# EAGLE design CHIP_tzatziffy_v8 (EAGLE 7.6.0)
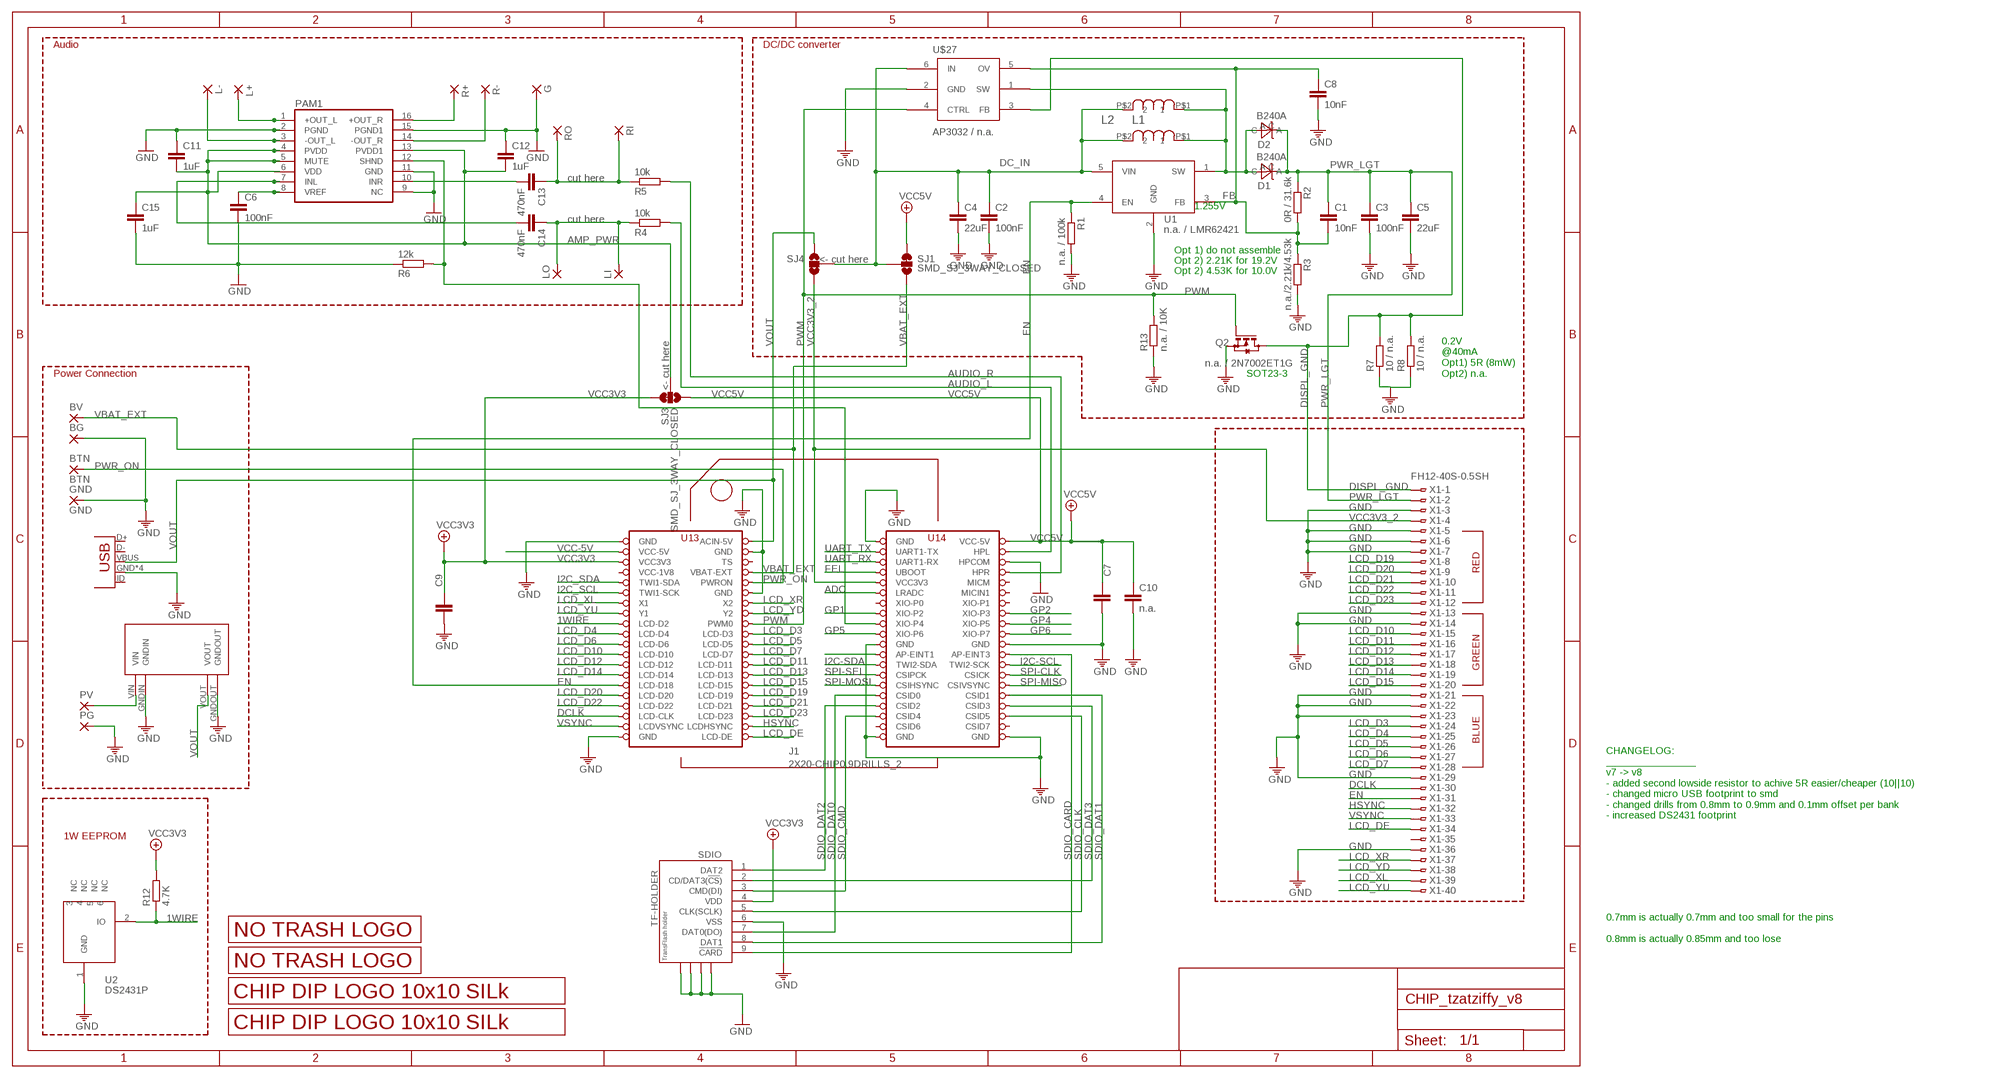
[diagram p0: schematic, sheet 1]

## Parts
BG  1,6/0,8  [1,6/0,8]
BTN  BTN  SMD2  [SMD1,27-2,54]
BV  1,6/0,8  [1,6/0,8]
C1  10nF  C-EUC0805  [C0805]
C2  100nF  C-EUC0805  [C0805]
C3  100nF  C-EUC0805  [C0805]
C4  22uF  C-EUC1206  [C1206]
C5  22uF  C-EUC1206  [C1206]
C6  100nF  C-EUC0805  [C0805]
C7  n.a.  C-EUC0805  [C0805]
C8  10nF  C-EUC0805  [C0805]
C9  n.a.  C-EUC0805  [C0805]
C10  n.a.  C-EUC0805  [C0805]
C11  1uF  C-EUC0805  [C0805]
C12  1uF  C-EUC0805  [C0805]
C13  470nF  C-EUC0805  [C0805]
C14  470nF  C-EUC0805  [C0805]
C15  1uF  C-EUC0805  [C0805]
D1  B240A  DIODE_SCHTKY_B240  [DO-214AC]
D2  B240A  DIODE_SCHTKY_B240  [DO-214AC]
G  1,6/0,8  [1,6/0,8]
GND  GND  SMD2  [SMD1,27-2,54]
J1  2X20-CHIP0.9DRILLS_2  [2X20CHIP_BANK_OFFSET_TH_0.9]
JP1  USBMICRO_SMD  [USB-B-MICRO-SMD_V03]
L1  SRN6045-100M  [SRN6045]
L2  SRN6045-100M  [SRN6045]
L+  1,6/0,8  [1,6/0,8]
L-  1,6/0,8  [1,6/0,8]
LI  1,6/0,8  [1,6/0,8]
LO  1,6/0,8  [1,6/0,8]
PAM1  PAM8403  [SOP-16]
PG  1,6/0,8  [1,6/0,8]
PV  1,6/0,8  [1,6/0,8]
Q2  n.a. / 2N7002ET1G  BSS123  [SOT23]
R1  n.a. / 100k  R-EU_M0805  [M0805]
R2  0R / 31.6k  R-EU_M0805  [M0805]
R3  n.a./2.21k/4.53k  R-EU_M0805  [M0805]
R4  10k  R-EU_R0805  [R0805]
R5  10k  R-EU_R0805  [R0805]
R6  12k  R-EU_R0805  [R0805]
R7  10 / n.a.  R-EU_M0805  [M0805]
R8  10 / n.a.  R-EU_M0805  [M0805]
R12  4.7K  R-EU_M0805  [M0805]
R13  n.a. / 10K  R-EU_M0805  [M0805]
R+  1,6/0,8  [1,6/0,8]
R-  1,6/0,8  [1,6/0,8]
RI  1,6/0,8  [1,6/0,8]
RO  1,6/0,8  [1,6/0,8]
SDIO  TF-HOLDER  [TF-PULL]
SJ1  SMD_SJ_3WAY_CLOSED  [SMD_SJ_3WAY_CLOSED]
SJ3  SMD_SJ_3WAY_CLOSED  [SMD_SJ_3WAY_CLOSED]
SJ4  SMD_SJ_3WAY_OPENT  [SMD_SJ_3WAY_OPEN]
U1  n.a. / LMR62421  LMR62421  [SOT23-5]
U2  DS2431P  [TSOC6]
U$2  LOGO_10X10_SILK  [LOGO2_10X10_SILK]
U$3  LOGO_NO_TRASHROHS  [LOGO_ROHS_SYM]
U$4  LOGO_NO_TRASHNO_TRASH  [LOGO_ROHS_NO_TRASH]
U$5  LOGO_10X10_SILK  [LOGO2_10X10_SILK]
U$10  MP1584EN_FRAMELESS  [MP1584EN_FRAMELESS]
U$27  AP3032 / n.a.  AP3032  [SOT23-6]
X1  FH12-40S-0.5SH  [FH12-40S-0.5SH]

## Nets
1WIRE: J1.LCD-D2 R12.1 U2.2(IO)
ADC: J1.LRADC
AMP_PWR: C11.2 C12.2 C15.1 PAM1.4(PVDD) PAM1.5(MUTE) PAM1.6(VDD) PAM1.13(PVDD1) SJ3.2
AUDIO_L: J1.HPL R4.2
AUDIO_R: J1.HPR R5.2
DC_IN: C2.1 C4.1 L1.P$2 L2.P$2 SJ1.2 SJ4.2 U1.5(VIN) U$27.6(IN)
DCLK: J1.LCD-CLK X1.30
DISPL_GND: Q2.3(D) R7.2 R8.2 U$27.3(FB) X1.1
EN: J1.LCD-D18 R1.1 U1.4(EN) X1.31
FB: C1.2 C8.1 R2.2 R3.1 U1.3(FB) U$27.5(OV)
FEL: J1.FEL(UBOOT)
GND: BG.1(P) C2.2 C3.2 C4.2 C5.2 C6.2 C7.2 C8.2 C9.2 C10.2 C11.1 C12.1 C15.2 G.1(P) GND.1(P) J1.GND@1(GND) J1.GND@2(GND) J1.GND@3(GND) J1.GND@4(GND) J1.GND@5(GND) J1.GND@6(GND) J1.GND@7(GND) J1.GND@8(GND) J1.GND@10(GND) J1.HPCOM JP1.GND JP1.SHIELD1(GND) JP1.SHIELD2(GND) JP1.SHIELD3(GND) PAM1.2(PGND) PAM1.9(NC) PAM1.11(GND) PAM1.15(PGND1) PG.1(P) Q2.2(S) R1.2 R3.2 R6.1 R7.1 R8.1 R13.1 SDIO.6(VSS) SDIO.S1 SDIO.S2 SDIO.S3 SDIO.S4 U1.2(GND) U2.1(GND) U$10.GNDIN U$10.GNDOUT U$27.2(GND) X1.3 X1.5 X1.6 X1.7 X1.13 X1.14 X1.21 X1.22 X1.23 X1.29 X1.36
GP1: J1.XIO-P2
GP2: J1.XIO-P3
GP3: J1.XIO-P4 PAM1.12(SHND) R6.2
GP4: J1.XIO-P5
GP5: J1.XIO-P6
GP6: J1.XIO-P7
HSYNC: J1.LCD-HSYNC(LCDHSYNC) X1.32
I2C-SCL: J1.TWI2-SCK
I2C-SDA: J1.TWI2-SDA
I2C_SCL: J1.TWI1-SCK
I2C_SDA: J1.TWI1-SDA
INL: C14.2 PAM1.7(INL)
INR: C13.2 PAM1.10(INR)
KPD_INT: J1.AP-EINT1
L+OUT: L+.1(P) PAM1.1(+OUT_L)
L-OUT: L-.1(P) PAM1.3(-OUT_L)
LCD_D3: J1.LCD-D3 X1.24
LCD_D4: J1.LCD-D4 X1.25
LCD_D5: J1.LCD-D5 X1.26
LCD_D6: J1.LCD-D6 X1.27
LCD_D7: J1.LCD-D7 X1.28
LCD_D10: J1.LCD-D10 X1.15
LCD_D11: J1.LCD-D11 X1.16
LCD_D12: J1.LCD-D12 X1.17
LCD_D13: J1.LCD-D13 X1.18
LCD_D14: J1.LCD-D14 X1.19
LCD_D15: J1.LCD-D15 X1.20
LCD_D19: J1.LCD-D19 X1.8
LCD_D20: J1.LCD-D20 X1.9
LCD_D21: J1.LCD-D21 X1.10
LCD_D22: J1.LCD-D22 X1.11
LCD_D23: J1.LCD-D23 X1.12
LCD_DE: J1.LCD-DE X1.34
LCD_XL: J1.X1 X1.39
LCD_XR: J1.X2 X1.37
LCD_YD: J1.Y2 X1.38
LCD_YU: J1.Y1 X1.40
N$38: C6.1 PAM1.8(VREF)
N$41: C14.1 LI.1(P) LO.1(P) R4.1
N$43: C13.1 R5.1 RI.1(P) RO.1(P)
PWM: J1.PWM0 Q2.1(G) R13.2 U$27.4(CTRL)
PWR_IN: PV.1(P) U$10.VIN
PWR_LGT: C1.1 C3.1 C5.1 D1.C D2.C R2.1 X1.2
PWR_ON: BTN.1(P) J1.PWRON
R+OUT: PAM1.16(+OUT_R) R+.1(P)
R-OUT: PAM1.14(-OUT_R) R-.1(P)
SDIO_CARD: J1.AP-EINT3 SDIO.9(!CARD)
SDIO_CLK: J1.CSID5 SDIO.5(CLK(SCLK))
SDIO_CMD: J1.CSID4 SDIO.3(CMD(DI))
SDIO_DAT0: J1.CSID0 SDIO.7(DAT0(DO))
SDIO_DAT1: J1.CSID1 SDIO.8(DAT1)
SDIO_DAT2: J1.CSID2 SDIO.1(DAT2)
SDIO_DAT3: J1.CSID3 SDIO.2(CD/DAT3(!CS!))
SPI-CLK: J1.CSICK
SPI-MISO: J1.CSIVSYNC
SPI-MOSI: J1.CSIHSYNC
SPI-SEL: J1.CSIPCK
UART_RX: J1.UART1-RX
UART_TX: J1.UART1-TX
VBAT_EXT: BV.1(P) J1.BAT(VBAT-EXT) SJ1.3
VCC3V3: C9.1 J1.VCC3V3 R12.2 SDIO.4(VDD) SJ3.1
VCC3V3_2: J1.VCC3V3@1(VCC3V3) SJ4.3 X1.4
VCC5V: C7.1 C10.1 J1.VCC5V@1(VCC-5V) SJ1.1 SJ3.3
VCC-5V: J1.VCC5V@0(VCC-5V)
VOUT: J1.CHG-IN(ACIN-5V) JP1.VBUS SJ4.1 U$10.VOUT
VREG_OUTPUT: D1.A D2.A L1.P$1 L2.P$1 U1.1(SW) U$27.1(SW)
VSYNC: J1.LCD-VSYNC(LCDVSYNC) X1.33
Unconnected: J1.CSID6 J1.CSID7 J1.MICIN1 J1.MICM J1.TS J1.XIO-P0 J1.XIO-P1 JP1.D+ JP1.D- JP1.ID U2.3(NC) U2.4(NC) U2.5(NC) U2.6(NC) X1.35

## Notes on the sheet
- Audio | DC/DC converter
- cut here
- 1.255V
- cut here
- Opt 1) do not assemble
- <- cut here | Opt 2) 2.21K for 19.2V
- Opt 2) 4.53K for 10.0V
- <- cut here
- Power Connection | SOT23-3
- 0.2V
  @40mA
  Opt1) 5R (8mW)
  Opt2) n.a.
- RED
- GREEN
- BLUE
- CHANGELOG:
  _______________
  v7 -> v8
  - added second lowside resistor to achive 5R easier/cheaper (10||10)
  - changed micro USB footprint to smd
  - changed drills from 0.8mm to 0.9mm and 0.1mm offset per bank
  - increased DS2431 footprint
- 1W EEPROM
- 0.7mm is actually 0.7mm and too small for the pins
  
  0.8mm is actually 0.85mm and too lose

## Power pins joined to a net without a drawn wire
VCC-1V8: J1.VCC1V8(VCC-1V8)

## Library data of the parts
BG BV G L+ L- LI LO PG PV R+ R- RI RO = wirepad:1,6/0,8: THROUGH-HOLE PAD
BTN GND = wirepad:SMD2: SMD PAD
C1-C15 = rcl:C-EU: CAPACITOR, European symbol
D1 D2 = Keyboard v0_5:DIODE_SCHTKY_B240; DESCRIPTION: DIODE SMD General Purpose 400V 1A 1.4W RoHS DO-214AC; FOOTPRINT: DO-214AC; LINK: http://www.digikey.com/product-detail/en/B240A-13-F/B240A-FDICT-ND/717810; MFG: DIGIKEY; MFG_PN: B240A-FDICT-ND; PART_TYPE: DIODE; PRICE: 0.11; VENDOR: DIODES; VENDOR_PART_NUMBER: B240A-13-F
J1 = JKW_CHIP:2X20-CHIP: Chip header; DESC: 0.9mm drills, moved outer rows 0.1mm towards outside, inner rows 0.1mm inwards
JP1 = JKW_CHIP:USB
L1 L2 = Keyboard v0_5:SRN6045-100M; DESCRIPTION: power inductor 10uH 2.5A 58.6 mohm; FOOTPRINT: SRN6045; LINK: http://www.digikey.com/product-detail/en/SRN6045-100M/SRN6045-100MTR-ND/2756120; MFG: DIGIKEY; MFG_PN: SRN6045-100MTR-ND; PART_TYPE: IND; PRICE: 0.15; TOLLERANCE: ±20%; VENDOR: BOURNS; VENDOR_PART_NUMBER: SRN6045-100M
PAM1 = JKW_CHIP:PAM8403: Dual channel audio amplifier IC - PAM8403
Q2 = transistor-small-signal:BSS123: N-CHANNEL MOS FET
R1-R8 R12 R13 = rcl:R-EU_: RESISTOR, European symbol
SDIO = JKW_CHIP:TF-HOLDER: TF / Micro SD socket is PUSH-PUSH type, the card can be pushed into and auto locked and pushed out by simply press the card. Surface Mounting type.
SJ1 SJ3 = JKW_CHIP:SMD_SJ_3WAY_CLOSED
SJ4 = JKW_CHIP:SMD_SJ_3WAY_OPEN: Solder Jumper 2 way solder jumper
U1 = PocketCHIP-Components-v0.7:LMR62421; DESCRIPTION: dc/dc step up, 2.1A, 1.6mhz, SOT-23-5; FOOTPRINT: SOT23-5; LINK: http://www.digikey.com/product-detail/en/LMR62421XMFE%2FNOPB/LMR62421XMFE%2FNOPBCT-ND/2777085; MFG: DIGIKEY; MFG_PN: LMR62421XMFE/NOPBCT-ND; PART_TYPE: IC; PRICE: 0.8; VENDOR: TEXAS INSTRUMENTS; VENDOR_PART_NUMBER: LMR62421XMFE/NOPB
U2 = JKW_CHIP:DS2431: 1024-Bit EEPROM This chip provides a 4x256 Bit EEPROM, which can be programmed@5V. Write protection and OTP emulation are available, too. Author: Jan Kandziora <jjj@gmx.de>; DESCRIPTION: IC, 1024-Bit, 1-Wire EEPROM, TSOC6; FOOTPRINT: TSOC6; LINK: http://www.digikey.com/product-detail/en/DS2431P%2BT%26R/DS2431P%2BT%26RCT-ND/3647900; MFG: DIGIKEY; MFG_PN: DS2431P+T&RCT-ND; PART_TYPE: IC; PRICE: 0.98; VENDOR: MAXIM; VENDOR_PART_NUMBER: DS2431P+T&R
U$2 U$5 = JKW_CHIP:LOGO_10X10_SILK
U$3 U$4 = JKW_CHIP:LOGO_NO_TRASH
U$10 = JKW_CHIP:MP1584EN_FRAMELESS
U$27 = JKW_CHIP:AP3032
X1 = Keyboard v0_5:FH12-40S-0.5S: 0.5mm Pitch Connectors For FPC/FFC Source: Data sheet; DESCRIPTION: CON ffc smd, bottom contact 40pos, 0.50mm R/A; FOOTPRINT: FH12-40S-0.5SH; LINK: http://www.digikey.com/product-detail/en/FH12-40S-0.5SH(55)/HFJ140CT-ND/1110388; MFG: DIGIKEY; MFG_PN: HFJ140CT-ND; VENDOR: HIROSE; VENDOR_PART_NUMBER: FH12-40S-0.5SH(55)

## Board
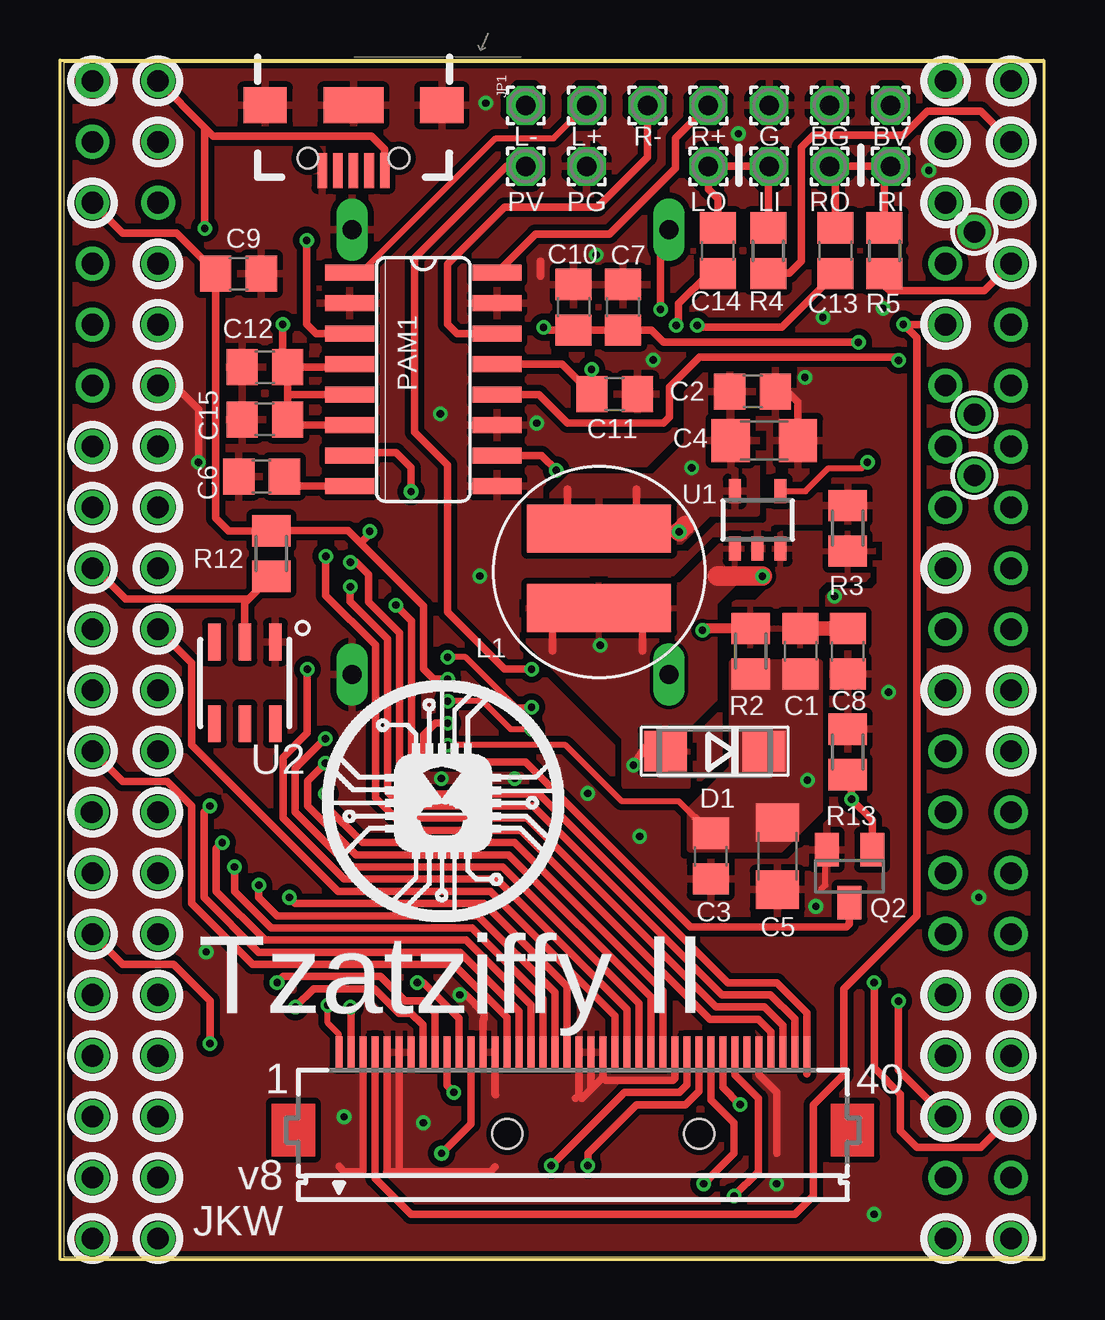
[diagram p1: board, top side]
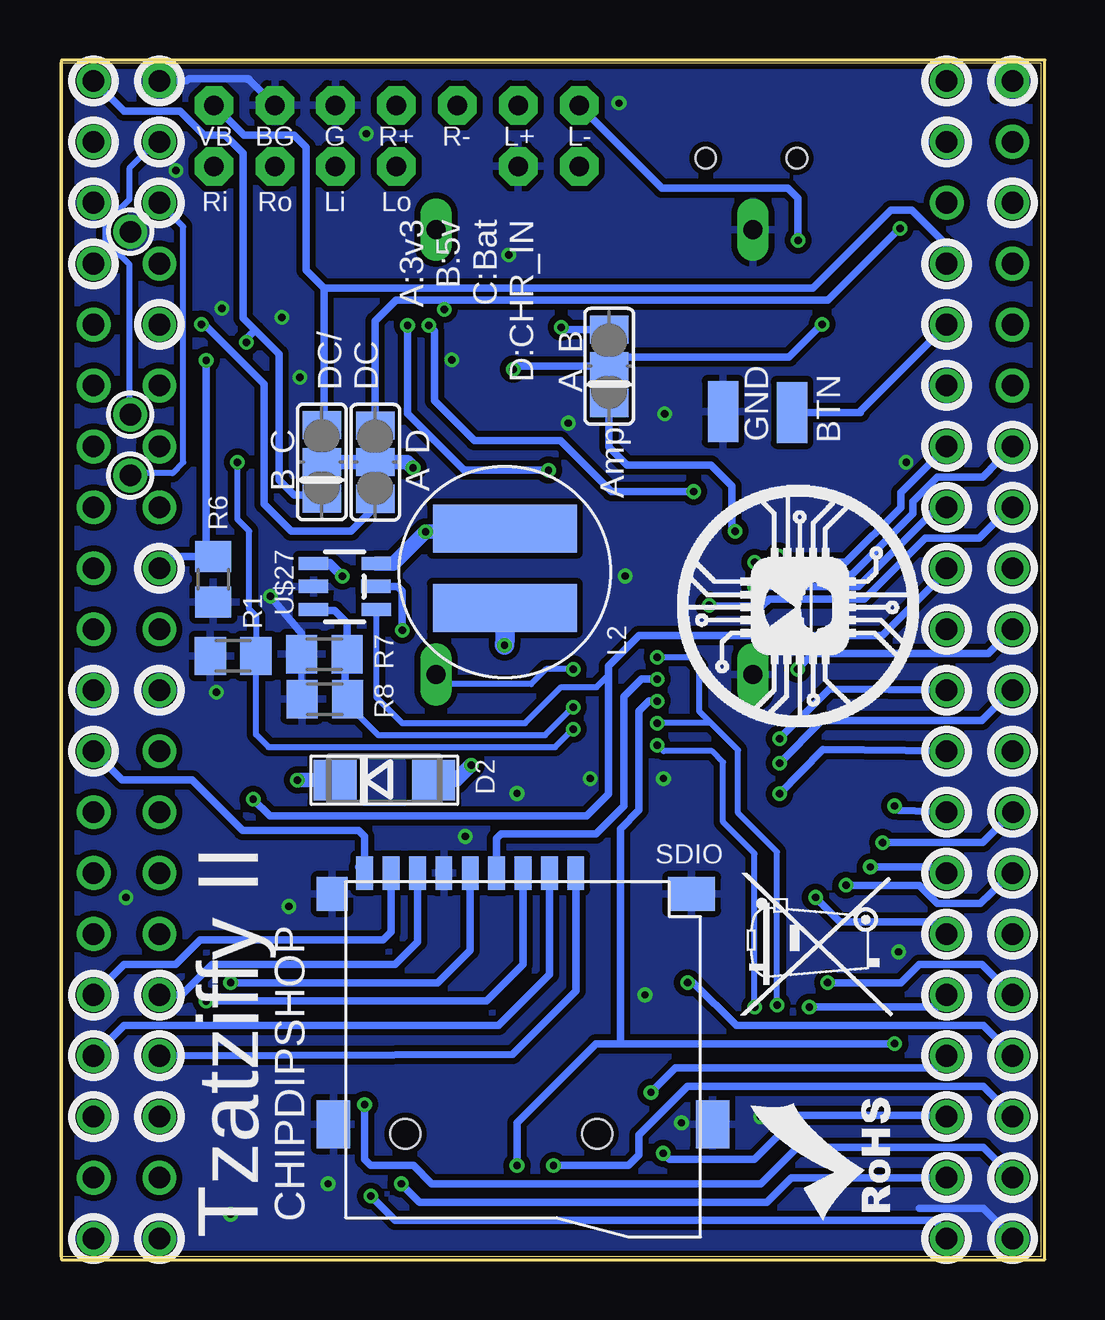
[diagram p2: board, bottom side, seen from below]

Size 41.05 x 50 mm. Coordinates in mm from the lower left corner, seen from the top.
Outline: 0.16,0.11 41.05,0.11 41.05,49.89 0.16,49.89 0.16,0.11
Copper layers (1*16): Top 0.035mm / dielectric 1.5mm / Bottom 0.035mm
Design rules "SeeedStudio_2layer_DRU_no_angle_20140221": minimum track width 6mil, minimum drill 12mil, track to track 6mil, track to pad 6mil, pad to pad 6mil, via to via 6mil, smd to smd 0mil, copper to edge 10mil, drill to drill 10mil, minimum pad ring 10mil, minimum via ring 6mil, stop-mask expansion 2mil, vias tented up to drill 100mil, thermal gap 10mil

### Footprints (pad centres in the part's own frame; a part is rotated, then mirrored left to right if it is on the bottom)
1,6/0,8 = drill 0.813 pad 1.6 octagon: 1 0,0
SMD1,27-2,54 = smd 1.27 x 2.54: 1 0,0
C0805 = smd 1.3 x 1.5: 1 -0.95,0; 2 0.95,0
C1206 = smd 1.6 x 1.8: 1 -1.4,0; 2 1.4,0
DO-214AC = smd 1.8 x 1.7: A 2.05,0; C -2.05,0
2X20CHIP_BANK_OFFSET_TH_0.9 = drill 0.9: AP-EINT1 15.14,-3.81; AP-EINT3 17.88,-3.81; BAT -17.68,16.51; CHG-IN -17.68,24.13; CSICK 17.88,-8.89; CSID0 15.14,-13.97; CSID1 17.88,-13.97; CSID2 15.14,-16.51; CSID3 17.88,-16.51; CSID4 15.14,-19.05; CSID5 17.88,-19.05; CSID6 15.14,-21.59; CSID7 17.88,-21.59; CSIHSYNC 15.14,-11.43; CSIPCK 15.14,-8.89; CSIVSYNC 17.88,-11.43; FEL 15.14,16.51; GND@1 -17.68,11.43; GND@2 -20.42,-24.13; GND@4 17.88,-1.27; GND@5 17.88,-24.13; GND@6 15.14,-24.13; GND@7 15.14,-1.27; GND@10 -17.68,21.59; HPCOM 17.88,19.05; HPL 17.88,21.59; HPR 17.88,16.51; LCD-CLK -20.42,-19.05; LCD-D2 -20.42,3.81; LCD-D3 -17.68,1.27; LCD-D4 -20.42,1.27; LCD-D5 -17.68,-1.27; LCD-D6 -20.42,-1.27; LCD-D7 -17.68,-3.81; LCD-D10 -20.42,-3.81; LCD-D11 -17.68,-6.35; LCD-D12 -20.447,-6.35; LCD-D13 -17.68,-8.89; LCD-D14 -20.42,-8.89; LCD-D15 -17.68,-11.43; LCD-D18 -20.42,-11.43; LCD-D19 -17.68,-13.97; LCD-D20 -20.42,-13.97; LCD-D21 -17.68,-16.51; LCD-D22 -20.42,-16.51; LCD-D23 -17.68,-19.05; LCD-DE -17.68,-24.13; LCD-HSYNC -17.68,-21.59; LCD-VSYNC -20.42,-21.59; LRADC 15.14,11.43; MICIN1 17.88,11.43; MICM 17.88,13.97; PWM0 -17.68,3.81; PWRON -17.68,13.97; TS -17.68,19.05; TWI1-SCK -20.42,11.43; TWI1-SDA -20.42,13.97; TWI2-SCK 17.88,-6.35; TWI2-SDA 15.14,-6.35; UART1-RX 15.14,19.05; UART1-TX 15.14,21.59; VCC1V8 -20.42,16.51; VCC3V3 -20.42,19.05; VCC3V3@1 15.14,13.97; VCC5V@0 -20.42,21.59; VCC5V@1 17.88,24.13; X1 -20.42,8.89; X2 -17.68,8.89; XIO-P0 15.14,8.89; XIO-P1 17.88,8.89; XIO-P2 15.14,6.35; XIO-P3 17.88,6.35; XIO-P4 15.14,3.81; XIO-P5 17.88,3.81; XIO-P6 15.14,1.27; XIO-P7 17.88,1.27; Y1 -20.42,6.35; Y2 -17.68,6.35 | drill 0.9 square: GND@3 -20.42,24.13; GND@8 15.14,24.13
USB-B-MICRO-SMD_V03 = smd 1.45 x 0.4: D+ 2.725,0; D- 2.725,0.65; GND 2.725,-1.3; ID 2.725,-0.65; VBUS 2.725,1.3 | smd 1.5 x 1.8: SHIELD1 0,3.685; SHIELD2 0,-3.685 | smd 1.5 x 2.5: SHIELD3 0,0 | hole 0.85: 2.2,1.9; 2.2,-1.9
SRN6045 = smd 2 x 6: P$1 1.5,0; P$2 -1.8,0
SOP-16 = smd 0.66 x 2.032: 1 -4.445,-3.073; 2 -3.175,-3.073; 3 -1.905,-3.073; 4 -0.635,-3.073; 5 0.635,-3.073; 6 1.905,-3.073; 7 3.175,-3.073; 8 4.445,-3.073; 9 4.445,3.073; 10 3.175,3.073; 11 1.905,3.073; 12 0.635,3.073; 13 -0.635,3.073; 14 -1.905,3.073; 15 -3.175,3.073; 16 -4.445,3.073
SOT23 = smd 1 x 1.4: 1 -0.95,-1.1; 2 0.95,-1.1; 3 0,1.1
M0805 = smd 1.3 x 1.6: 1 -0.95,0; 2 0.95,0
R0805 = smd 1.3 x 1.5: 1 -0.95,0; 2 0.95,0
TF-PULL = smd 0.7 x 1.4: 1 -2.2,-7.62; 2 -1.1,-7.62; 3 0,-7.62; 4 1.1,-7.62; 5 2.2,-7.62; 6 3.3,-7.62; 7 4.4,-7.62; 8 5.5,-7.62; 9 6.6,-7.62 | smd 1.4 x 2: S1 -7.9,2.85; S2 7.9,2.85 | smd 1.28 x 1.4: S3 7.96,-6.75 | smd 1.95 x 1.4: S4 -7.025,-6.75 | hole 1.25: -3.1,3.25; 4.9,3.25
SMD_SJ_3WAY_CLOSED = smd 1.168 x 1.6: 1 -1.524,0; 2 0,0; 3 1.524,0
SMD_SJ_3WAY_OPEN = smd 1.168 x 1.6: 1 -1.524,0; 2 0,0; 3 1.524,0
SOT23-5 = smd 0.5 x 1: 1 -0.95,-1.2; 2 0,-1.2; 3 0.95,-1.2; 4 0.95,1.2; 5 -0.95,1.2
TSOC6 = smd 0.53 x 1.53: 1 -1.27,-1.7; 2 0,-1.7; 3 1.27,-1.7; 4 1.27,1.7; 5 0,1.7; 6 -1.27,1.7
MP1584EN_FRAMELESS = drill 0.8 long: GNDIN 1.778,14.986; GNDOUT 20.32,14.986; VIN 1.778,1.778; VOUT 20.32,1.778
SOT23-6 = smd 0.559 x 1.219: 1 -0.95,-1.3; 2 0,-1.3; 3 0.965,-1.3; 4 0.965,1.321; 5 0,1.3; 6 -0.95,1.321
FH12-40S-0.5SH = smd 0.3 x 1.3: 1 -9.75,3.25; 2 -9.25,3.25; 3 -8.75,3.25; 4 -8.25,3.25; 5 -7.75,3.25; 6 -7.25,3.25; 7 -6.75,3.25; 8 -6.25,3.25; 9 -5.75,3.25; 10 -5.25,3.25; 11 -4.75,3.25; 12 -4.25,3.25; 13 -3.75,3.25; 14 -3.25,3.25; 15 -2.75,3.25; 16 -2.25,3.25; 17 -1.75,3.25; 18 -1.25,3.25; 19 -0.75,3.25; 20 -0.25,3.25; 21 0.25,3.25; 22 0.75,3.25; 23 1.25,3.25; 24 1.75,3.25; 25 2.25,3.25; 26 2.75,3.25; 27 3.25,3.25; 28 3.75,3.25; 29 4.25,3.25; 30 4.75,3.25; 31 5.25,3.25; 32 5.75,3.25; 33 6.25,3.25; 34 6.75,3.25; 35 7.25,3.25; 36 7.75,3.25; 37 8.25,3.25; 38 8.75,3.25; 39 9.25,3.25; 40 9.75,3.25

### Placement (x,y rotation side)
BG  32.09,48.11 0 top
BTN  10.54,35.31 180 bottom
BV  34.63,48.11 0 top
C1  30.87,25.36 90 top
C2  28.87,36.18 0 top
C3  27.13,16.82 270 top
C4  29.36,34.14 0 top
C5  29.91,16.82 270 top
C6  8.41,32.64 180 top
C7  23.47,39.7 90 top
C8  32.83,25.36 270 top
C9  7.45,41.09 0 top
C10  21.41,39.7 90 top
C11  23.13,36.07 180 top
C12  8.54,37.19 0 top
C13  32.33,42.05 270 top
C14  27.42,42.05 270 top
C15  8.54,35.02 180 top
D1  27.29,21.18 180 top
D2  27.54,19.98 0 bottom
G  29.57,48.11 0 top
GND  13.41,35.35 180 bottom
J1  21.77,25 0 top
JP1  12.23,48.11 270 top
L1  22.48,28.66 270 top
L2  22.51,28.66 270 bottom
L+  21.95,48.11 0 top
L-  19.41,48.11 0 top
LI  29.57,45.57 0 top
LO  27.03,45.57 0 top
PAM1  15.15,36.68 270 top
PG  21.95,45.57 0 top
PV  19.41,45.57 0 top
Q2  32.91,15.98 180 top
R1  33.83,25.16 180 bottom
R2  28.79,25.36 90 top
R3  32.83,30.48 90 top
R4  29.53,42.05 270 top
R5  34.37,42.05 270 top
R6  34.66,28.36 90 bottom
R7  30.04,25.23 0 bottom
R8  30.01,23.36 0 bottom
R12  8.81,29.43 90 top
R13  32.83,21.16 270 top
R+  27.03,48.11 0 top
R-  24.49,48.11 0 top
RI  34.63,45.57 0 top
RO  32.09,45.57 0 top
SDIO  21.75,8.49 180 bottom
SJ1  30.14,33.25 90 bottom
SJ3  18.16,37.23 90 bottom
SJ4  27.91,33.23 270 bottom
U1  29.08,30.83 0 top
U2  7.71,24.04 180 top
U$2  10.95,14.08 0 top
U$3  6.37,1.19 90 bottom
U$4  6.33,10.13 90 bottom
U$5  5.26,22.21 90 bottom
U$10  27.16,22.61 90 top
U$27  29.19,28.06 270 bottom
X1  21.38,5.39 0 top

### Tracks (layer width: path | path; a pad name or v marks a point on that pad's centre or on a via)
1WIRE
  Top 0.305: 7.87,27.54 2.74,27.54 1.47,28.81 J1.LCD-D2 | 7.87,27.54 R12.1 | 7.87,27.54 7.71,27.37 U2.2
AMP_PWR  (via drill 0.3)
  Top 0.305: 9.62,37.32 C12.2 | PAM1.6 10.13,34.78 C15.1 9.49,35.98 | C12.2 9.49,35.98 | PAM1.4 11.95,37.19 C12.2 | v9.29,38.98 9.29,37.4 C12.2 | 18.18,37.36 PAM1.13 20.93,37.32 C11.2 21.78,35.85 22.16,36.23 v22.16,37.11 | PAM1.5 9.56,36.05 9.49,35.98
  Bottom 0.305: v9.29,38.98 10.66,37.61 17.79,37.61 SJ3.2 22.04,37.23 v22.16,37.11
AUDIO_L
  Top 0.305: 29.16,40.98 29.15,40.99 R4.2 29.16,41.11 30.41,41.11 30.91,41.61 30.91,46.36 31.41,46.86 35.16,46.86 36.16,47.86 38.38,47.86 J1.HPL
AUDIO_R
  Top 0.305: R5.2 34.35,40.61 34.58,40.38 38.52,40.38 J1.HPR
DC_IN  (via drill 0.3)
  Top 0.305: 21.16,32.11 21.16,31.11 | 24.04,32.11 24.04,31.11
  Top 0.813: v25.81,30.33 26.07,30.59
  Bottom 0.61: 22.68,29.88 22.48,30.08 22.51,30.08 L2.P$2 22.64,30.33 v25.81,30.33 27.14,29.01 U$27.6 | SJ1.2 27.93,33.25 | 27.93,33.25 SJ4.2 | 27.93,33.25 26.58,33.25 v26.33,33
  pour Top: 29.04,36.86 26.91,36.86 26.16,36.11 26.16,33.98 24.79,32.61 21.29,32.61 19.66,30.98 19.66,29.61 25.54,29.61 27.04,31.11 29.04,31.11
DCLK  (via drill 0.3)
  Top 0.305: X1.30 26.13,7.28 25.81,6.97 23.53,6.97 v20.48,3.92
  Bottom 0.305: v20.48,3.92 17.35,3.92 16.91,4.36 16.91,5.2 14.89,7.22 2.56,7.22 1.35,6.01 J1.LCD-CLK
DISPL_GND  (via drill 0.3)
  Top 0.254: X1.1 11.63,9.39 11.16,9.86 v11.16,10.61 | v16.16,25.11 16.91,25.11 18.99,23.03 v19.66,23.03
  Top 0.305: v16.16,22.36 15.66,22.36 15.16,21.86 15.16,21.11 15.54,20.73 19.41,20.73 26.29,13.86 32.78,13.86 32.91,13.98 Q2.3
  Bottom 0.254: v11.16,10.61 11.16,16.98 12.79,18.61 12.79,21.23 13.91,22.36 | 13.91,22.36 v16.16,22.36 | v16.16,25.11 14.79,25.11 14.41,24.73 14.41,22.86 13.91,22.36 | 30.54,27.05 U$27.3 | 29.16,23.23 27.79,21.86 20.83,21.86 v19.66,23.03 | R8.2 29.16,23.36
  Bottom 0.305: 29.16,23.23 29.16,23.36 29.16,25.16 R7.2 29.09,26.53 29.6,27.05 30.54,27.05
EN  (via drill 0.3)
  Top 0.254: v16.16,23.28 17.62,23.28 18.79,22.11 v19.66,22.11 | U1.4 31.08,32.03 32.03,32.98 33.41,32.98 v33.66,33.23
  Top 0.305: X1.31 26.63,7.02 26.07,6.46 24.04,6.46 22,4.43 v22,3.92 | v6.26,9 6.26,10.78 4.73,12.3 2.62,12.3 J1.LCD-D18
  Bottom 0.254: v33.66,33.23 33.66,30.86 33.16,30.36 33.16,27.11 32.89,26.83 R1.1 | 32.53,25.06 R1.1 | v19.66,22.11 20.41,21.36 32.36,21.36 32.89,21.88 R1.1
  Bottom 0.305: v6.26,9 17.69,9 | 17.69,9 17.69,17.96 16.91,18.73 16.91,22.86 16.49,23.28 v16.16,23.28 | 17.69,9 18.7,9 22,5.7 v22,3.92
FB  (via drill 0.3)
  Top 0.406: R2.2 26.86,26.31 v26.79,26.23
  Top 0.61: C8.1 C1.2
  Bottom 0.305: U$27.5 26.99,28.06 26.79,27.86 v26.79,26.23
  pour Top: 28.04,26.23 28.16,25.61 31.54,25.61 31.54,27.98 31.91,28.36 33.53,28.36 33.91,28.73 33.91,30.11 33.78,30.23 30.04,30.23 29.79,29.98 29.79,28.11 29.04,27.36 28.16,27.36 28.04,27.23
GND  (via drill 0.3, 0.9 pad 1.42)
  Top 0.254: 31.72,15.42 31.91,15.61 31.91,16.53 Q2.2
  Top 0.305: 14.13,3.66 17.94,3.66 18.13,3.86 | PAM1.2 12.2,39.99 | 11.63,3.88 11.84,3.66 12.61,3.66 12.63,3.69 X1.3 | 14.13,3.66 13.62,3.66 13.63,3.67 X1.5 | X1.6 14.13,3.67 14.13,3.66 | X1.36 29.13,7.71 29.88,6.97 29.88,4.43 | 16.92,11.03 17.69,10.27 17.69,10.01 17.63,9.96 X1.13 | X1.29 25.63,7.55 25.56,7.47 22.75,7.47 22.63,7.59 | X1.21 21.63,6.85 21.5,6.71 | X1.23 22.63,7.59 | 22.63,7.59 22.13,7.09 | 22.13,7.09 21.75,6.71 | X1.22 22.13,7.09 | X1.14 18.13,6.89 18.16,6.86 | C4.2 30.76,35.74 30.32,36.18 C2.2 | 20.04,40.98 20.04,41.61 | J1.GND@1 4.79,36.43 5.79,35.43 5.79,33.24 v5.78,33.23
  Bottom 0.254: R8.1 30.98,23.38 R7.1
  Bottom 0.305: 5.24,2.14 2.56,2.14 1.35,0.93 J1.GND@2 | 33.17,49.19 33.24,49.19 | BG.1 33.22,49.23 35.66,49.23 35.7,49.19 35.76,49.13 J1.GND@8 | R7.1 30.98,26.1 v32.29,27.65
  other vias: 24.73,37.51 17.5,28.49 17.75,48.2 22,19.43 33.94,1.89 29.88,3.16 24.16,17.64 38.3,15.09 18.96,20.05 15.9,20.05 15.15,5.7 16.67,11.03 11.84,5.95 38.12,42.84 34.54,23.65 31.05,36.77 19.87,34.86 28.28,46.93 6.09,12.83 22.35,41.88 15.85,35.26 31.8,39.27 34.31,39.65 36.22,45.4 31.51,14.72
  pour Bottom (isolate 0.254, rank 3): 0.67,49.89 40.29,49.89 40.29,0.36 0.67,0.36
  pour Top (isolate 0.254, rank 3): 0.67,49.89 40.29,49.89 40.29,0.36 0.67,0.36
GP3  (via drill 0.3)
  Top 0.305: v34.96,37.48 34.83,37.61 26.66,37.61 25.41,36.36 25.41,35.11 25.16,34.86 21.16,34.86 19.97,36.05 PAM1.12
  Bottom 0.305: v34.96,37.48 34.96,29.61 R6.2 36.41,29.31 J1.XIO-P4
HSYNC  (via drill 0.3)
  Top 0.305: 27.13,3.46 v26.83,3.16 28.1,4.42 28.1,5.7 27.13,6.66 X1.32
  Bottom 0.305: v26.83,3.16 26.07,2.39 11.59,2.39 10.57,3.41 J1.LCD-HSYNC 3.96,3.41
INL  (via drill 0.3)
  Top 0.305: PAM1.7 12.2,33.64 14.01,33.64 14.63,33.01 v14.63,32.01 | v25.68,38.94 25.79,39.05 25.79,39.84 27.04,41.1 C14.2
  Bottom 0.305: v14.63,32.01 18.06,32.01 20.2,34.14 23.78,34.14 25.43,35.79 25.43,38.69 v25.68,38.94
INR  (via drill 0.3)
  Top 0.305: v26.56,38.94 26.65,38.86 30.09,38.86 C13.2 | PAM1.10 20.08,33.51 v20.69,32.9
  Bottom 0.305: v26.56,38.94 26.56,35.26 24.2,32.9 v20.69,32.9
L+OUT
  Top 0.254: L+.1 20.57,46.73 18.16,46.73 12.56,41.13 PAM1.1
  Top 0.305: PAM1.1 12.66,41.13
L-OUT  (via drill 0.3)
  Top 0.305: PAM1.3 10.68,38.59 10.29,38.98 v10.29,42.48
  Bottom 0.305: v10.29,42.48 10.29,44.23 10.71,44.66 15.96,44.66 L-.1
LCD_D3
  Top 0.305: X1.24 23.13,10.16 17.94,15.35 11.59,15.35 5.49,21.44 5.49,24.87 J1.LCD-D3
LCD_D4  (via drill 0.3)
  Top 0.305: X1.25 23.63,10.42 18.19,15.86 11.84,15.86 9.3,18.4 9.3,20.93 10.31,21.94 v10.31,24.61
  Bottom 0.305: v10.31,24.61 9.66,25.25 2.37,25.25 J1.LCD-D4
LCD_D5  (via drill 0.3)
  Top 0.305: X1.26 24.13,10.68 18.45,16.36 12.1,16.36 9.81,18.65 9.81,20.46 v11.06,21.71
  Bottom 0.305: v11.06,21.71 8.98,23.79 J1.LCD-D5
LCD_D6  (via drill 0.3)
  Top 0.305: X1.27 24.63,10.94 18.7,16.87 12.35,16.87 10.32,18.9 10.32,19.95 v11.06,20.69
  Bottom 0.305: v11.06,20.69 9.29,22.46 2.62,22.46 J1.LCD-D6
LCD_D7  (via drill 0.3)
  Top 0.305: X1.28 25.13,11.2 18.96,17.38 12.61,17.38 11.08,18.9 v11.06,19.41
  Bottom 0.305: v11.06,19.41 9.24,21.25 J1.LCD-D7
LCD_D10
  Top 0.305: X1.15 18.63,10.08 16.42,12.3 8.03,12.3 5.49,14.84 5.49,18.9 4.48,19.92 2.62,19.92 J1.LCD-D10
LCD_D11  (via drill 0.3)
  Top 0.305: v6.26,18.9 6,18.65 6,15.09 8.29,12.81 16.67,12.81 19.13,10.35 X1.16
  Bottom 0.305: v6.26,18.9 6.06,18.71 J1.LCD-D11
LCD_D12  (via drill 0.3)
  Top 0.305: v6.76,17.38 6.51,17.13 6.51,15.35 8.54,13.32 16.92,13.32 19.63,10.61 X1.17
  Bottom 0.305: v6.76,17.38 2.59,17.38 J1.LCD-D12
LCD_D13  (via drill 0.3)
  Top 0.305: v7.27,16.36 7.27,15.35 8.8,13.82 17.18,13.82 20.13,10.87 X1.18
  Bottom 0.305: v7.27,16.36 4.34,16.36 J1.LCD-D13
LCD_D14  (via drill 0.3)
  Top 0.305: X1.19 20.63,11.13 17.43,14.33 9.05,14.33 8.29,15.09 v8.29,15.6
  Bottom 0.305: v8.29,15.6 5.24,15.6 4.48,14.84 2.69,14.84 J1.LCD-D14
LCD_D15  (via drill 0.3)
  Top 0.305: X1.20 21.13,11.39 17.69,14.84 9.81,14.84 v9.56,15.09
  Bottom 0.305: v9.56,15.09 8.54,14.08 4.6,14.08 J1.LCD-D15
LCD_D19  (via drill 0.3)
  Top 0.305: X1.8 15.13,9.77 14.64,10.27 14.13,10.27 13.11,11.28 10.57,11.28 v9.81,10.52
  Bottom 0.305: v9.81,10.52 4.46,10.52 4.09,10.9 J1.LCD-D19
LCD_D20  (via drill 0.3)
  Top 0.305: X1.9 15.63,10.29 15.15,10.78 14.38,10.78 13.37,11.79 9.3,11.79 v9.05,11.54
  Bottom 0.305: v9.05,11.54 6,11.54 5.24,12.3 2.62,12.3 J1.LCD-D20
LCD_D21  (via drill 0.3)
  Top 0.305: v16.42,6.97 16.13,7.25 X1.10
  Bottom 0.305: v16.42,6.97 15.4,7.98 4.52,7.98 4.09,8.41 J1.LCD-D21
LCD_D22  (via drill 0.3)
  Top 0.305: X1.11 16.63,10.05 15.15,11.54 v14.89,11.54
  Bottom 0.305: v14.89,11.54 14.64,11.54 12.86,9.76 2.56,9.76 1.35,8.54 J1.LCD-D22
LCD_D23  (via drill 0.3)
  Top 0.305: 17.13,8.28 X1.12 17.13,5.65 v15.91,4.43
  Bottom 0.305: v15.91,4.43 15.65,4.17 12.1,4.17 10.26,6.01 4.15,6.01 J1.LCD-D23
LCD_DE  (via drill 0.3)
  Top 0.305: X1.34 28.13,7.7 29.12,6.71 29.12,3.66 v28.1,2.65
  Bottom 0.305: v28.1,2.65 27.08,1.63 4.6,1.63 4.09,1.13 J1.LCD-DE
LCD_XL  (via drill 0.3)
  Top 0.305: v12.1,29.06 12.35,29.06 12.86,28.56 12.86,27.41 14.16,26.11 14.16,19.73 14.99,18.9 19.72,18.9 27.59,11.03 29.62,11.03 30.63,10.02 X1.39
  Bottom 0.305: v12.1,29.06 11.59,28.56 8.03,28.56 5.49,31.1 5.49,31.6 4.48,32.62 2.59,32.62 J1.X1
LCD_XR  (via drill 0.3)
  Top 0.305: X1.37 29.63,9.5 29.12,10.01 27.08,10.01 19.21,17.89 14.51,17.89 13.16,19.23 13.16,25.61 11.08,27.69 v11.08,29.32
  Bottom 0.305: v11.08,29.32 10.83,29.06 8.29,29.06 6,31.35 6,31.98 J1.X2
LCD_YD  (via drill 0.3)
  Top 0.305: X1.38 30.13,9.76 29.37,10.52 27.34,10.52 19.46,18.4 14.75,18.4 13.66,19.48 13.66,25.86 12.1,27.42 v12.1,28.05
  Bottom 0.305: v12.1,28.05 7.78,28.05 4.48,31.35 J1.Y2
LCD_YU  (via drill 0.3)
  Top 0.305: 31.13,7.74 X1.40 31.13,10.28 29.88,11.54 27.85,11.54 19.97,19.41 15.23,19.41 14.66,19.98 14.66,26.62 v14,27.28
  Bottom 0.305: v14,27.28 13.95,27.23 11.79,27.23 11.48,27.54 7.53,27.54 4.99,30.08 2.74,30.08 1.47,31.35 J1.Y1
N$38
  Top 0.305: C6.1 9.76,32.24 PAM1.8
N$41
  Top 0.305: C14.1 27.42,44.22 27.03,44.61 LO.1 LI.1 29.53,45.52 R4.1
N$43
  Top 0.305: RO.1 RI.1 34.37,45.31 R5.1 | 32.08,45.55 RO.1 | C13.1 32.33,45.33 RO.1
PWM  (via drill 0.3)
  Top 0.305: Q2.1 33.86,18.32 v33,19.18 33,20.04 R13.2
  Bottom 0.254: 32.85,19.16 v33,19.18 | U$27.4 27.87,23.44 26.79,22.36 21.66,22.36 20.16,23.86 18.69,23.86 18.19,24.36
  Bottom 0.305: v33,19.18 32.3,18.48 19.11,18.48 18.19,19.41 18.19,24.36 18.19,24.75 16.92,26.02 6.76,26.02 4.09,28.69 J1.PWM0
PWR_IN  (via drill 0.3)
  Top 0.305: PV.1 18.62,45.57 14.79,41.73 14.79,34.48 16.16,33.11 16.16,26.98 18.54,24.61 v19.66,24.61
  Bottom 0.254: 25.1,24.11 U$10.VIN 24.98,23.98 21.41,23.98 20.79,24.61 v19.66,24.61
PWR_LGT  (via drill 0.3)
  Top 0.254: 26.72,18.17 25.79,19.11 23.41,19.11 21.08,21.44 v16.16,21.44
  Top 0.305: X1.2 12.13,10.49 v12.1,10.52 | 26.47,18.42 26.72,18.17 C3.1
  Bottom 0.254: v12.1,10.52 12.1,16.92 13.41,18.23 13.41,20.72 13.88,21.19 15.89,21.19 v16.16,21.44
  Bottom 0.61: D2.C v31.16,19.98
  pour Top (no thermals): 28.04,24.86 31.66,24.86 31.66,18.73 30.04,17.11 26.29,17.11 26.29,18.73 28.04,20.48
PWR_ON
  Bottom 0.305: BTN.1 7.69,35.31 7.69,35.37 J1.PWRON
R+OUT
  Top 0.254: 18.43,41.13 PAM1.16
  Top 0.305: 18.56,41.13 PAM1.16 19.82,42.73 22.91,42.73 25.66,45.48 25.66,46.73 R+.1
R-OUT
  Top 0.305: PAM1.14 16.55,38.59 16.16,38.98 16.16,41.48 18.54,43.86 22.41,43.86 24.49,45.94 R-.1
SDIO_CARD
  Bottom 0.305: 28.61,16.37 SDIO.9 28.35,17.63 28.61,17.89 33.43,17.89 35.55,20 38.46,20 J1.AP-EINT3
SDIO_CLK  (via drill 0.3)
  Top 0.305: v33.94,11.54 33.94,7.98 35.03,6.89 35.03,5.36 35.71,4.68 38.38,4.68 J1.CSID5
  Bottom 0.305: SDIO.5 23.95,12.89 25.31,11.54 v33.94,11.54
SDIO_CMD  (via drill 0.3)
  Top 0.305: v34.96,10.78 34.96,7.9 J1.CSID4
  Bottom 0.305: SDIO.3 21.75,12.3 23.27,10.78 v34.96,10.78
SDIO_DAT0
  Bottom 0.305: SDIO.7 26.15,13.23 27.08,12.3 34.7,12.3 35.97,11.03 J1.CSID0
SDIO_DAT1
  Bottom 0.305: SDIO.8 27.25,13.66 27.59,13.32 35.21,13.32 36.23,12.3 38.38,12.3 J1.CSID1
SDIO_DAT2
  Bottom 0.305: SDIO.1 19.55,11.2 22.2,8.55 J1.CSID2
SDIO_DAT3
  Bottom 0.305: SDIO.2 20.65,11.88 22.77,9.76 38.38,9.76 J1.CSID3
UART_RX  (via drill 0.9 pad 1.42)
  Bottom 0.254: v38.12,32.68 38.06,32.78 36.36,32.78 35.91,33.23 35.91,43.05 J1.UART1-RX
UART_TX  (via drill 0.9 pad 1.42)
  Bottom 0.22: 38.16,44.18 39.16,43.17 | 39.16,42.48 38.16,41.48
  Bottom 0.254: 38.16,44.18 38.16,45.48 37.05,46.59 J1.UART1-TX | 39.16,43.17 39.16,42.48 | 38.16,41.48 38.16,35.26 v38.12,35.22
VBAT_EXT
  Bottom 0.305: SJ1.3 30.05,34.86 30.05,37.46 30.04,37.48 30.04,40.48 | 30.04,40.48 9.66,40.48 6.41,43.73 5.54,43.73 4.09,42.29 J1.BAT | BV.1 33.38,46.86 31.29,46.86 30.79,46.36 30.79,41.23 30.04,40.48
VCC3V3  (via drill 0.3)
  Top 0.305: 8.54,30.65 R12.2 | 6.26,41.33 C9.1 | 9.02,30.59 R12.2 | 8.8,30.39 R12.2 | 6.47,41.11 C9.1 | C9.1 6.5,41.15 4.86,42.78 2.62,42.78 J1.VCC3V3 | 12.54,29.86 12.02,30.38 R12.2 | R12.2 8.79,30.36 7.04,30.36 6.5,30.9 C9.1 | v12.91,30.36 12.91,30.23 12.54,29.86 | v16.16,24.19 15.57,24.19 15.16,24.61 15.16,27.23 12.54,29.86
  Bottom 0.305: SDIO.4 22.85,17.54 22.66,17.73 18.72,17.73 17.55,18.9 17.55,23.47 16.82,24.19 v16.16,24.19 | v12.91,30.36 13.04,30.48 13.04,32.23 13.91,33.11 17.41,33.11 18.16,33.86 SJ3.1
VCC3V3_2  (via drill 0.3)
  Top 0.305: X1.4 13.13,3.39 14.64,1.89 30.64,1.89 31.4,2.65 31.4,6.46 32.67,7.73 32.67,11.28 35.72,14.33 35.72,38.42 v35.16,38.98 35.17,38.97 J1.VCC3V3@1
  Bottom 0.305: v35.16,38.98 35.03,38.98 32.53,36.48 32.53,31.48 31.41,30.36 28.91,30.36 27.91,31.36 SJ4.3
VCC5V  (via drill 0.3)
  Top 0.305: v20.16,38.86 20.27,38.75 C10.1 C7.1 24.65,38.75 25.16,38.23 v33.28,38.23
  Bottom 0.305: 30.16,31.7 SJ1.1 30.27,31.86 31.29,31.86 31.91,32.48 31.91,37.73 32.91,38.73 | 19.93,38.76 v20.16,38.86 20.06,38.76 SJ3.3 | v33.28,38.23 33.28,38.36 32.91,38.73 | 32.91,38.73 33.41,39.23 33.41,46.11 34.16,46.86 35.03,46.86 36.03,47.86 38.38,47.86 J1.VCC5V@1
VOUT  (via drill 0.3)
  Top 0.305: v6.04,42.98 6.04,47.19 | v25.04,39.61 25.04,42.58 U$10.VOUT | 6.04,47.19 J1.CHG-IN | 6.04,47.19 6.39,46.83 12.98,46.83 13.54,46.28 JP1.VBUS
  Bottom 0.305: SJ4.1 27.91,39.11 27.04,39.98 25.04,39.98 | v6.04,42.98 9.04,39.98 25.04,39.98 | v25.04,39.61 25.04,39.98
VREG_OUTPUT  (via drill 0.3)
  Top 0.305: v23.91,20.61 24.41,21.36 | 20.54,26.61 20.54,25.36 | 24.29,26.61 24.29,25.36
  Top 0.813: v29.29,28.48 27.41,28.48
  Bottom 0.406: U$27.1 29.81,29.01 v29.29,28.48
  Bottom 0.61: D2.A 24.54,19.98 v23.91,20.61
  Bottom 0.813: L2.P$1 22.51,25.87 v22.52,25.61
  pour Top: 19.54,28.11 25.91,28.11 27.79,29.98 28.41,29.98 28.41,28.48 27.29,27.36 27.29,23.36 26.16,22.23 26.16,19.73 23.54,19.73 23.54,21.73 19.54,25.73
VSYNC  (via drill 0.3)
  Top 0.305: X1.33 27.63,7.18 v28.35,6.46
  Bottom 0.305: v28.35,6.46 28.35,4.17 28.1,3.92 26.32,3.92 25.56,3.16 11.84,3.16 10.32,4.68 2.56,4.68 1.35,3.47 J1.LCD-VSYNC

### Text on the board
tNames: Tzatziffy II | 1 | 40 | v8 / JKW
bNames: L- | L+ | R- | R+ | G | BG | VB | Lo | Li | Ro | Ri | A:3v3 / B:5v / C:Bat / D:CHR_IN | B | A | DC/ / DC | D | C | A | B | Amp | CHIPDIPSHOP | Tzatziffy II

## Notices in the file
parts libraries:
JKW_CHIP: License : http://creativecommons.org/licenses/by-sa/3.0
(Creative Commons 3.0)
